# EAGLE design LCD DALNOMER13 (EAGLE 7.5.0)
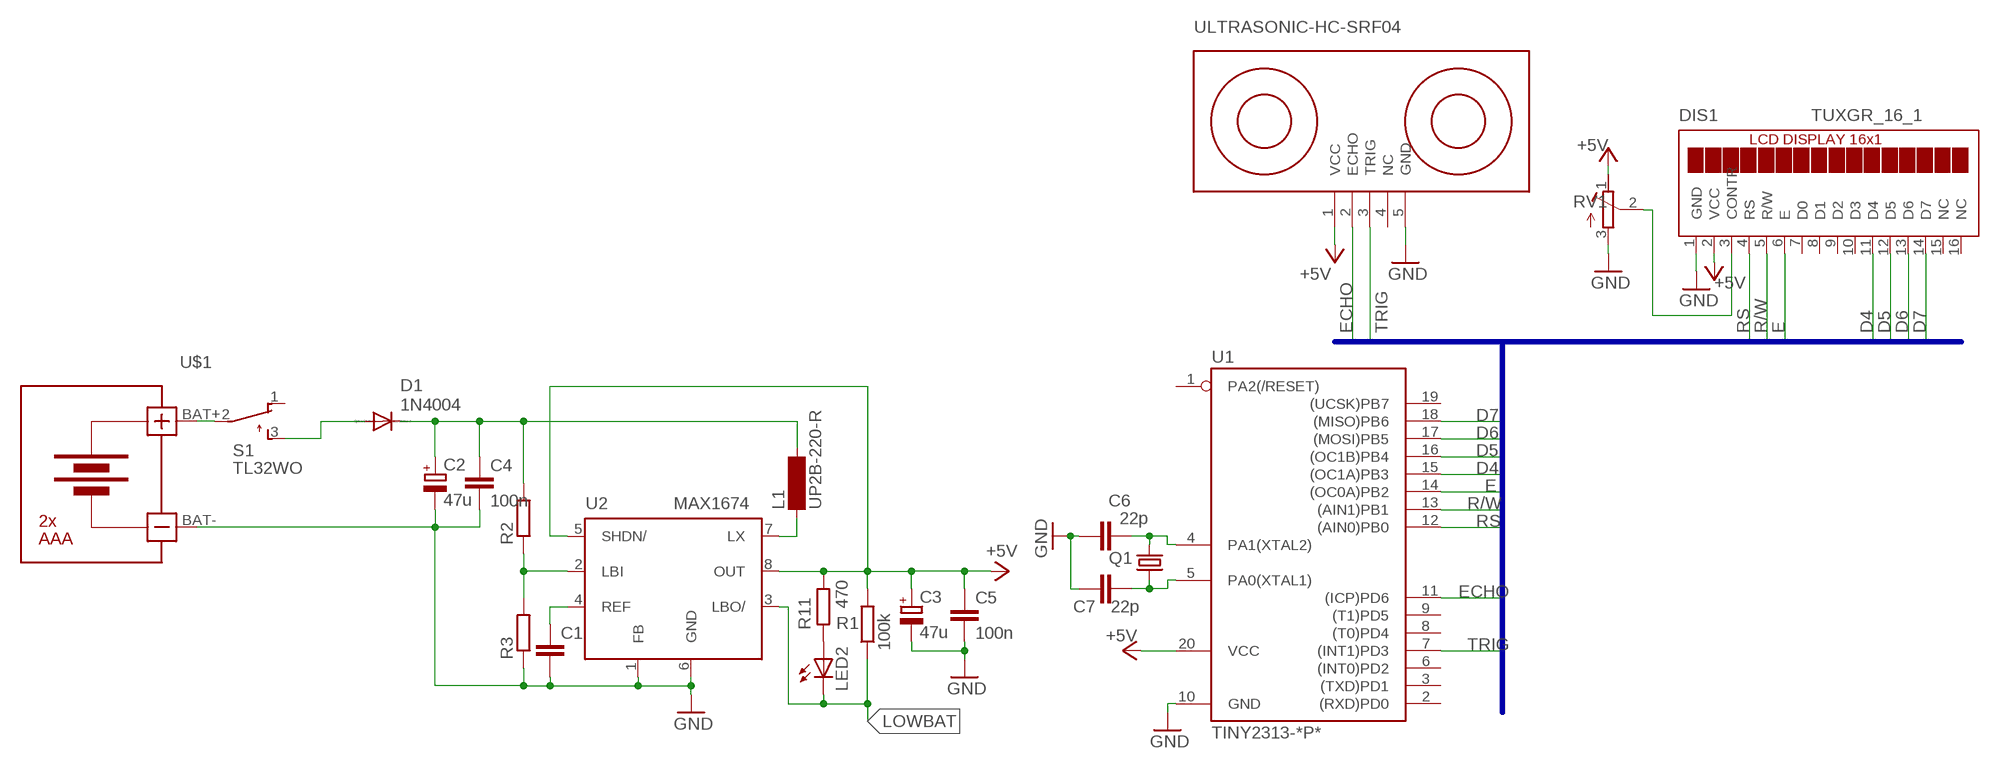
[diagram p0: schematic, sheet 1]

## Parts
C1  C-EUC1206  [C1206]
C2  47u  CPOL-EUSMCB  [SMC_B]
C3  47u  CPOL-EUSMCB  [SMC_B]
C4  100n  C-EUC1206  [C1206]
C5  100n  C-EUC1206  [C1206]
C6  22p  C-EUC1206  [C1206]
C7  22p  C-EUC1206  [C1206]
D1  1N4004  [DO41-10]
DIS1  TUXGR_16_1  [TUXGR_16X1]
L1  UP2B-220-R  MS85  [MS85]
LED2  LED3MM  [LED3MM]
Q1  CRYSTALHC49UP  [HC49UP]
R1  100k  R-EU_R1206  [R1206]
R2  R-EU_R1206  [R1206]
R3  R-EU_R1206  [R1206]
R11  470  R-EU_R1206  [R1206]
RV1  R-TRIMM-3386-F  [R-TRIMM-3386F]
S1  TL32WO  [TL3XWO]
SONAR1  ULTRASONIC-HC-SRF04  [ULTRASONIC-SRF04]
U1  TINY2313-*P*  [DIL20]
U2  MAX1674  [UMAX8]
U$1  BATTERY-HOLDER-2AAA  [BATTERY-HOLDER-2AAA]

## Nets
+5V: C3.+ C5.1 DIS1.2(VCC) R1.2 R11.1 RV1.1(A) SONAR1.1(VCC) U1.20(VCC) U2.5(SHDN/) U2.8(OUT)
D4: DIS1.11(D4) U1.15((OC1A)PB3)
D5: DIS1.12(D5) U1.16((OC1B)PB4)
D6: DIS1.13(D6) U1.17((MOSI)PB5)
D7: DIS1.14(D7) U1.18((MISO)PB6)
E: DIS1.6(E) U1.14((OC0A)PB2)
ECHO: SONAR1.2(ECHO) U1.11((ICP)PD6)
GND: C1.2 C2.- C3.- C4.2 C5.2 C6.1 C7.1 DIS1.1(GND) R3.1 RV1.3(E) SONAR1.5(GND) U1.10(GND) U2.1(FB) U2.6(GND) U$1.BAT-
LOWBAT: LED2.K(C) R1.1 U2.3(LBO/)
N$1: L1.1 U2.7(LX)
N$2: C2.+ C4.1 D1.C L1.2 R2.2
N$3: R2.1 R3.2 U2.2(LBI)
N$4: LED2.A R11.2
N$5: DIS1.3(CONTR) RV1.2(S)
N$6: C6.2 Q1.2 U1.4(PA1(XTAL2))
N$7: C1.1 U2.4(REF)
N$8: C7.2 Q1.1 U1.5(PA0(XTAL1))
N$16: S1.2(P) U$1.BAT+
N$17: D1.A S1.3(S)
R/W: DIS1.5(R/W) U1.13((AIN1)PB1)
RS: DIS1.4(RS) U1.12((AIN0)PB0)
TRIG: SONAR1.3(TRIG) U1.7((INT1)PD3)
Unconnected: DIS1.7(D0) DIS1.8(D1) DIS1.9(D2) DIS1.10(D3) DIS1.15(NC) DIS1.16(NC) S1.1(O) SONAR1.4(NC) U1.1(PA2(/RESET)) U1.2((RXD)PD0) U1.3((TXD)PD1) U1.6((INT0)PD2) U1.8((T0)PD4) U1.9((T1)PD5) U1.19((UCSK)PB7)

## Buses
B$1

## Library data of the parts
C1 C4-C7 = rcl:C-EU: CAPACITOR, European symbol
C2 C3 = rcl:CPOL-EU: POLARIZED CAPACITOR, European symbol
D1 = diode:1N4004: DIODE
DIS1 = display-lcd:TUXGR_16_1: 1x16 LCD DISPLAY
L1 = inductor-neosid:MS85: INDUCTOR; OC_FARNELL: unknown; OC_NEWARK: unknown
LED2 = led:LED: LED
Q1 = crystal:CRYSTAL: CRYSTAL; OC_FARNELL: unknown; OC_NEWARK: unknown
R1-R3 R11 = rcl:R-EU_: RESISTOR, European symbol
RV1 = rcl:R-TRIMM-3386-F
S1 = switch:TL32WO: TINY SWITCH ON - MOM Source: http://www2.produktinfo.conrad.com/datenblaetter/700000-724999/705152-da-01-de-Subminiaturschalter_TL_36WO.pdf
SONAR1 = diy-modules:ULTRASONIC-HC-SRF04
U1 = avr-7:TINY2313*: Atmel Tiny2313 2K Flash, 128 bytes EEPROM, 128 bytes RAM
U2 = maxim:MAX1674: DC/DC CONVERTER; MF: MAXIM; MPN: MAX1674EUA+; OC_FARNELL: 1379864; OC_NEWARK: 23K5719
U$1 = diy-modules:BATTERY-HOLDER-2AAA: Battery Holder 2 x AAA

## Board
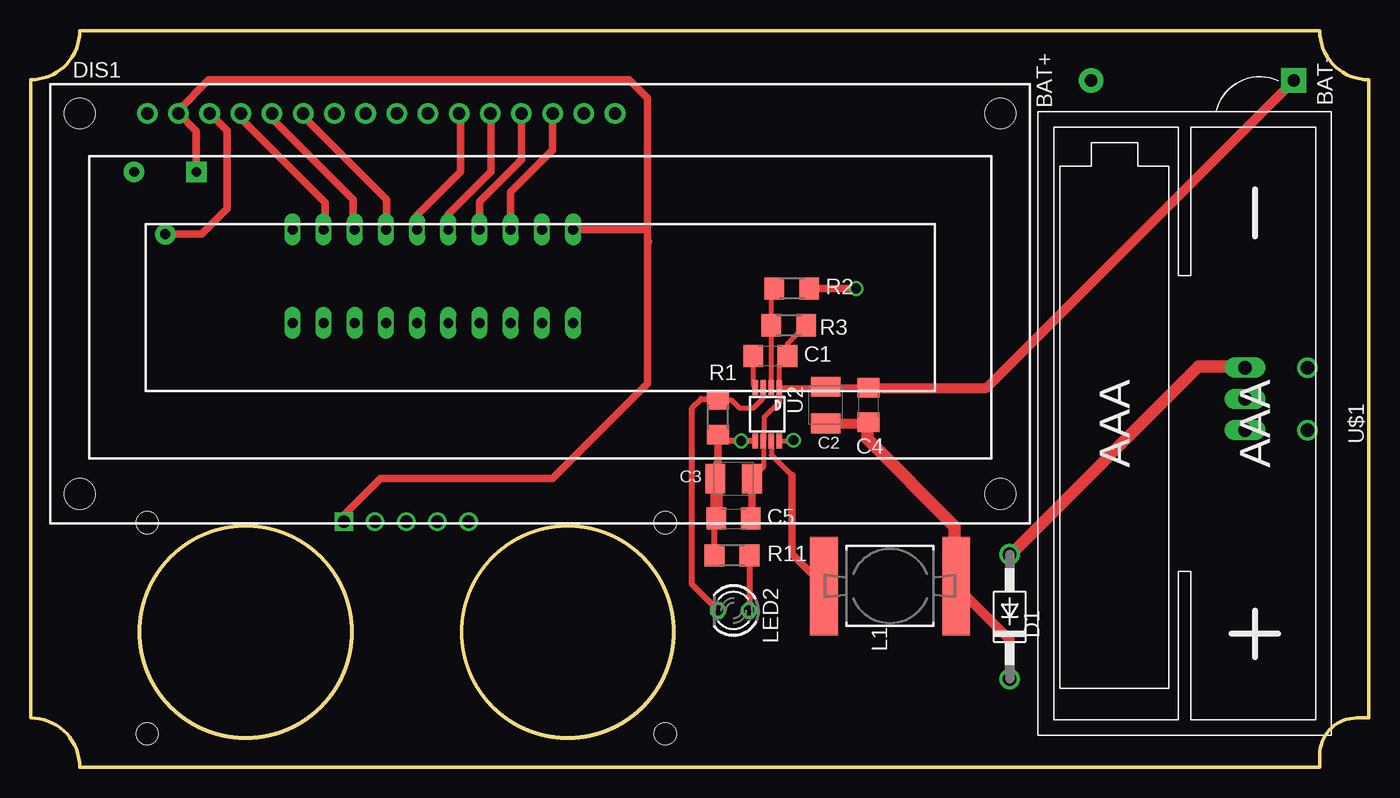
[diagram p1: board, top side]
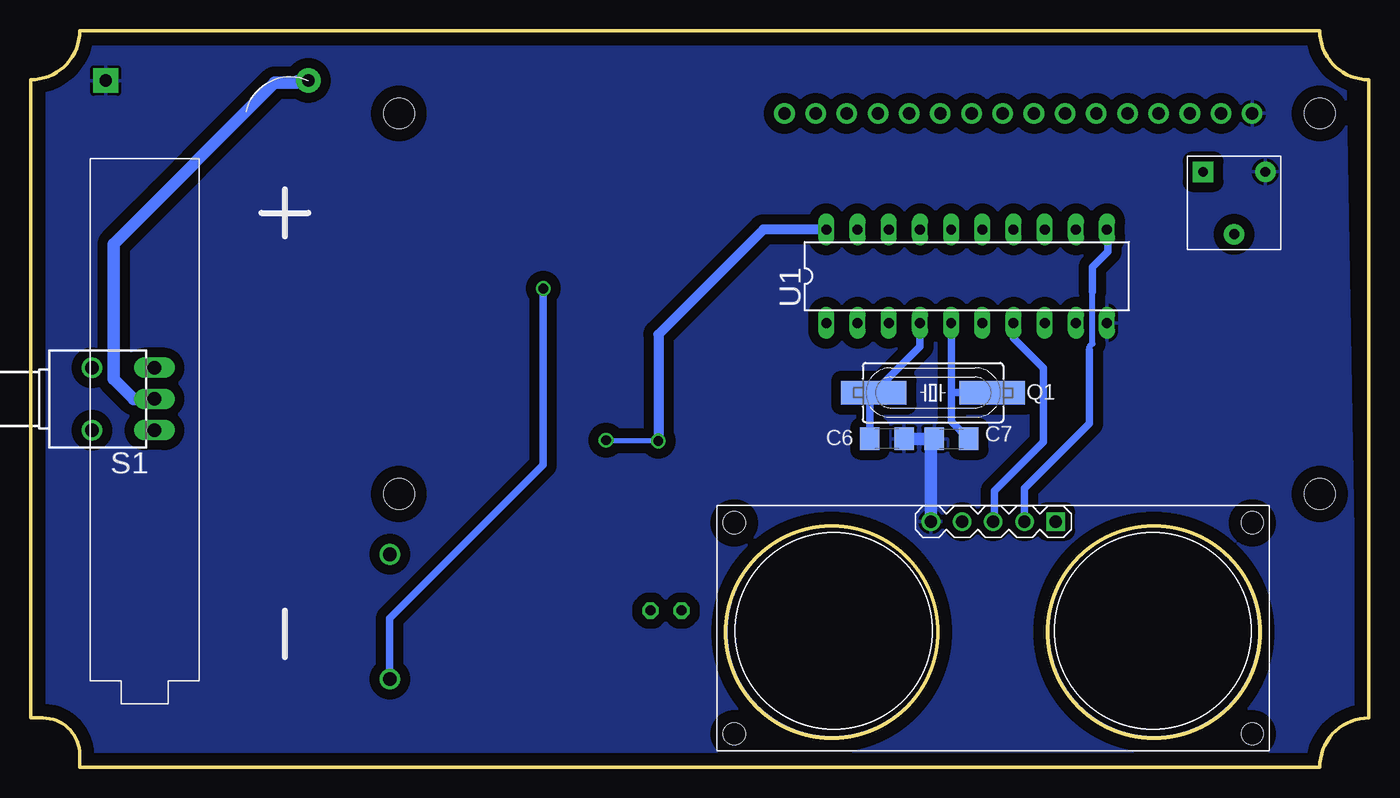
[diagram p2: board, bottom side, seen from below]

Size 109 x 60 mm. Coordinates in mm from the lower left corner, seen from the top.
Outline: 105,0 4,0 arc90 0,4 0,56 arc90 4,60 105,60 arc90 109,56 109,4 108,4 arc90 105,1 105,0
Outline: circle at 17.5,11 radius 8.63
Outline: circle at 43.75,11 radius 8.63
Copper layers (1*16): Top 0.035mm / dielectric 1.5mm / Bottom 0.035mm
Design rules "default": minimum track width 10mil, minimum drill 24mil, track to track 8mil, track to pad 8mil, pad to pad 8mil, via to via 8mil, smd to smd 8mil, copper to edge 40mil, drill to drill 8mil, minimum pad ring 10mil, minimum via ring 8mil, stop-mask expansion 4mil, vias tented up to drill 0mil, thermal gap 10mil
Holes 17 mm at 17.5,11 43.75,11

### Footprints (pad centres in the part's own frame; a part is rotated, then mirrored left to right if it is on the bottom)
C1206 = smd 1.6 x 1.8: 1 -1.4,0; 2 1.4,0
SMC_B = smd 1.6 x 2.4: + -1.5,0; - 1.5,0
DO41-10 = drill 1.118: A 5.08,0; C -5.08,0
TUXGR_16X1 = drill 1 pad 1.676: 1 -0.25,0.26; 2 2.29,0.26; 3 4.83,0.26; 4 7.37,0.26; 5 9.91,0.26; 6 12.45,0.26; 7 14.99,0.26; 8 17.53,0.26; 9 20.07,0.26; 10 22.61,0.26; 11 25.15,0.26; 12 27.69,0.26; 13 30.23,0.26; 14 32.77,0.26; 15 35.31,0.26; 16 37.85,0.26 | hole 2.5: -5.75,-30.74; 69.25,-30.74; -5.75,0.26; 69.25,0.26
MS85 = smd 8 x 2.25: 1 0,-5.383; 2 0,5.383
LED3MM = drill 0.813 octagon: A -1.27,0; K 1.27,0
HC49UP = smd 5.334 x 1.93: 1 -4.826,0; 2 4.826,0
R1206 = smd 1.6 x 1.803: 1 -1.422,0; 2 1.422,0
R-TRIMM-3386F = drill 0.8 pad 1.676 square: 1 0,0 | drill 0.8 pad 1.676: 2 5.08,2.54; 3 0,5.08
TL3XWO = drill 1.1 pad 1.422 long: 1 -2.54,-5.08; 2 0,-5.08; 3 2.54,-5.08 | drill 1.1 pad 1.676: M1 -2.54,0; M2 2.54,0
ULTRASONIC-SRF04 = drill 1 square: 1 16.51,0 | drill 1: 2 19.05,0; 3 21.59,0; 4 24.13,0; 5 26.67,0 | hole 1.8: 0.49,17.29; 0.49,0.09; 42.69,0.09; 42.69,17.29
DIL20 = drill 0.813 long: 1 -11.43,-3.81; 2 -8.89,-3.81; 3 -6.35,-3.81; 4 -3.81,-3.81; 5 -1.27,-3.81; 6 1.27,-3.81; 7 3.81,-3.81; 8 6.35,-3.81; 9 8.89,-3.81; 10 11.43,-3.81; 11 11.43,3.81; 12 8.89,3.81; 13 6.35,3.81; 14 3.81,3.81; 15 1.27,3.81; 16 -1.27,3.81; 17 -3.81,3.81; 18 -6.35,3.81; 19 -8.89,3.81; 20 -11.43,3.81
UMAX8 = smd 0.45 x 1.2: 1 -0.975,-2.175; 2 -0.325,-2.175; 3 0.325,-2.175; 4 0.975,-2.175; 5 0.975,2.175; 6 0.325,2.175; 7 -0.325,2.175; 8 -0.975,2.175
BATTERY-HOLDER-2AAA = drill 1 pad 2: BAT+ -27.94,-7.62 | drill 1 pad 2 square: BAT- -27.94,8.89

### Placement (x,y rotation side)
C1  60.25,33.5 0 top
C2  64.75,29.5 90 top
C3  57.25,23.5 0 top
C4  68.25,29.5 90 top
C5  57.25,20.25 0 top
C6  39.25,26.75 180 bottom
C7  34,26.75 0 bottom
D1  79.75,12.25 90 top
DIS1  9.75,53 0 top
L1  70,14.75 270 top
LED2  57.25,12.75 180 top
Q1  35.5,30.5 180 bottom
R1  56,28.5 270 top
R2  62,39 0 top
R3  61.75,36 180 top
R11  57.12,17.25 0 top
RV1  13.5,48.5 270 bottom
S1  104,30 90 bottom
SONAR1  9,20 180 bottom
U1  32.75,40 0 bottom
U2  60,28.75 180 top
U$1  94,28 270 top

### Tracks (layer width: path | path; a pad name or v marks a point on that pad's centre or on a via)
+5V  (via drill 0.8)
  Top 0.406: U2.8 62.08,26.57 v62.12,26.62
  Top 0.5: U2.5 v57.88,26.57 56.5,26.57 R1.2 | R11.1 55.7,20.1 C5.1
  Top 0.61: R1.2 56,23.75 C3.+ | 55.75,20.15 C5.1 | SONAR1.1 25.51,20.51 28.5,23.5 42.5,23.5 50.25,31.25 50.25,42.75 | 50.25,43.75 50.25,54.5 48.75,56 14.5,56 12.04,53.54 DIS1.2 13.5,51.8 RV1.1 | 50.25,43.75 50.25,42.75 | 50.25,42.75 50.31,42.81 | U1.20 50.19,43.81 50.25,43.75
  Top 1.016: C5.1 55.85,23.4 C3.+
  Bottom 0.406: v62.12,26.62 57.92,26.62 v57.88,26.57
  Bottom 0.813: U1.20 49.31,43.81 57.88,35.25 v57.88,26.57
D4
  Top 0.61: U1.15 31.48,44.98 35,48.5 35,53.16 DIS1.11
D5
  Top 0.61: U1.16 34.02,45.02 37.5,48.5 37.5,53.2 DIS1.12
D6
  Top 0.61: U1.17 36.56,46.06 40,49.5 40,53.24 DIS1.13
D7
  Top 0.61: U1.18 39.1,46.85 42.5,50.25 42.5,53.24 DIS1.14
E
  Top 0.61: DIS1.6 22.2,53.05 29,46.25 29,43.87 U1.14
ECHO
  Bottom 0.5: 22.75,34 22.75,34.25 22.5,34.5 22.5,38.75
  Bottom 0.61: SONAR1.2 28.05,22.7 22.75,28 22.75,34 | 22.5,38.75 22.5,40.75 21.25,42 21.25,43.74 U1.11
GND
  Top 0.406: U2.1 60.98,32.83 C1.2 61.65,34.48 R3.1 | U2.1 64.67,30.93 C2.- 68.15,31 C4.2 | C3.- 59.67,24.43 U2.6 59.75,26.65 59.75,28.5 60.98,29.73 U2.1
  Top 0.61: C3.- 58.75,20.35 C5.2
  Top 0.813: C4.2 77.85,30.9 U$1.BAT-
  Bottom 1.016: SONAR1.5 35.67,26.48 C7.1 C6.1
  pour Bottom (isolate 0.813): 108,59 108,0.5 1,0.5 2,58.75
LOWBAT
  Top 0.406: R1.1 57.08,29.92 57.75,29.25 58.88,29.25 59.62,30 59.62,30.88 U2.3
  Top 0.5: LED2.K 55.98,12.77 53.88,14.88 53.88,29.25 54.62,30 55.92,30 R1.1
N$1
  Top 0.406: U2.7 60.33,25.43 62,23.75
  Top 0.61: 62,23.75 62,17.37 L1.1
N$2  (via drill 0.8)
  Top 0.61: R2.2 v67.25,39
  Top 0.813: D1.C 79.75,10.38 L1.2 | 63.55,39.12 R2.2 | C2.+ 68.15,28 C4.1
  Top 1.016: 68.15,28 68.15,26.73 75.25,19.62 75.25,14.88 L1.2
  Bottom 0.61: v67.25,39 67.25,24.62 79.75,12.12 D1.C
N$3
  Top 0.406: U2.2 R3.2 60.33,38.75 R2.1
N$4
  Top 0.5: R11.2 58.55,12.78 LED2.A
N$5
  Top 0.61: RV1.2 13.92,43.42 16,45.5 16,51.84 DIS1.3
N$6
  Bottom 0.61: U1.4 36.56,34.27 Q1.2 40.65,30.18 C6.2
N$7
  Top 0.406: C1.1 58.85,31.1 U2.4
N$8
  Bottom 0.61: U1.5 34.02,30.5 | 34.02,30.5 34.02,28.17 C7.2 | Q1.1 34.02,30.5
N$16
  Bottom 1.016: S1.2 100.62,30 102.25,31.62 102.25,42.62 89.12,55.75 87.38,55.75 87.25,55.88 86.44,55.88 U$1.BAT+
N$17
  Top 1.016: D1.A 79.83,17.33 95.12,32.62 98.83,32.62 S1.3
R/W
  Top 0.61: DIS1.5 19.66,52.84 26.25,46.25 26.25,43.96 U1.13
RS
  Top 0.61: DIS1.4 17.12,52.88 24,46 24,43.95 U1.12
TRIG
  Bottom 0.61: U1.7 28.94,34.94 26.5,32.5 26.5,26.5 30.5,22.5 30.5,20.09 SONAR1.3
